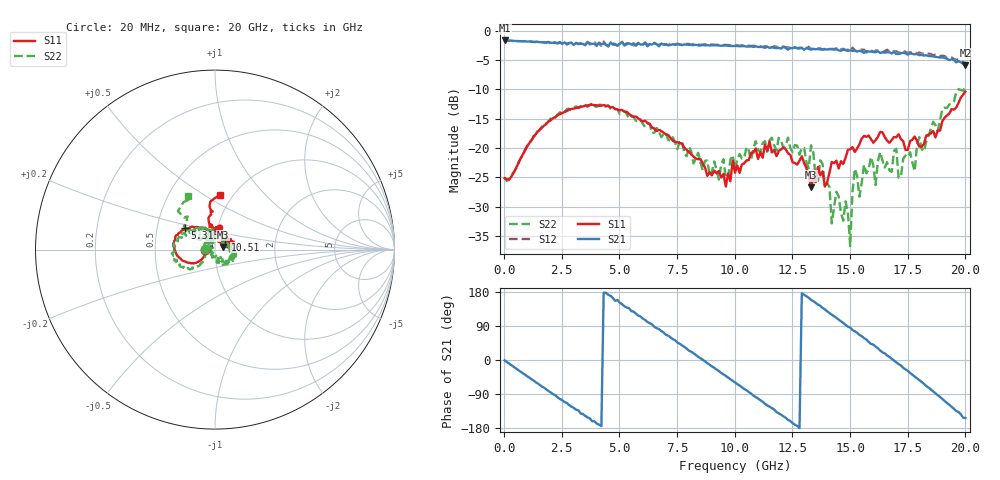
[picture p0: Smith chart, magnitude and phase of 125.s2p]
!Agilent Technologies,N5230A,US43500223,A.07.50.48
!Agilent N5230A: A.07.50.48
!Date: Sunday, September 13, 2015 22:02:00
!Correction: S11(Full 2 Port(1,2))
!S21(Full 2 Port(1,2))
!S12(Full 2 Port(1,2))
!S22(Full 2 Port(1,2))
!S2P File: Measurements: S11, S21, S12, S22:
# Hz S  dB  R 50
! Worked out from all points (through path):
!   201 points, 20 MHz to 20 GHz, reference 50 ohm
!   highest |S21| = -1.65 dB at 20 MHz (marker M1); lowest = -5.9 dB at 20 GHz (marker M2)
!   group delay of S21, straight-line fit = 120 ps
!   lowest |S11| = -26.7 dB at 13.31 GHz (marker M3), VSWR 1.10, Z = 54.6 + j1.55 ohm
!   |S11| at or under -10 dB: start of sweep to end of sweep
!   |S22| runs from -36.7 to -9.6 dB; largest |S21 - S12| = 0.051
!   S11 on the Smith chart (normalised r, x): 20 MHz: 0.89, +0.00; 5.315 GHz: 0.70, +0.17; 10.51 GHz: 1.11, +0.13; 20 GHz: 0.87, +0.58
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2e7  -25.12 179.9  -1.65 -1.0  -1.67 -1.0  -24.97 179.0
1.9181e9  -15.48 -154.2  -1.90 -81.6  -1.91 -82.0  -15.49 -140.4
3.4166e9  -12.92 177.7  -2.25 -142.6  -2.51 -141.9  -12.62 -164.9
5.3147e9  -13.80 144.6  -2.32 138.5  -2.12 140.1  -14.17 151.4
6.7133e9  -16.90 120.6  -2.66 81.6  -2.47 80.8  -17.12 118.1
8.3117e9  -21.80 101.3  -2.38 13.4  -2.26 13.2  -21.71 88.6
1.001e10  -24.20 58.4  -2.59 -59.2  -2.45 -59.8  -23.57 6.5
1.05095e10  -22.11 45.7  -2.71 -80.2  -2.59 -81.7  -19.81 2.8
1.21079e10  -19.90 15.4  -2.75 -148.8  -2.67 -148.8  -19.99 -26.8
1.33067e10  -26.68 17.9  -3.21 158.9  -3.12 158.1  -19.55 -49.8
1.34066e10  -24.92 31.4  -3.10 155.4  -3.06 154.7  -20.75 -68.6
1.41059e10  -24.21 60.8  -3.15 123.8  -3.11 122.0  -26.61 -110.8
1.42058e10  -22.38 58.2  -3.16 119.7  -3.09 120.1  -32.84 -138.3
1.48052e10  -21.63 68.0  -3.33 92.7  -3.28 91.5  -29.08 -163.7
1.5005e10  -20.21 62.4  -3.35 85.3  -3.44 86.0  -36.72 139.6
1.52048e10  -20.66 65.4  -3.41 75.7  -3.28 73.7  -23.53 153.5
1.54046e10  -19.36 73.4  -3.41 66.3  -3.20 68.1  -28.29 102.7
1.59041e10  -18.48 74.6  -3.54 42.4  -3.29 43.6  -21.53 110.2
1.67033e10  -19.10 83.7  -3.67 8.1  -3.57 6.1  -23.78 113.6
1.78022e10  -18.02 87.0  -4.03 -44.0  -3.66 -45.8  -23.93 141.8
1.85015e10  -17.51 96.8  -4.34 -77.3  -3.94 -80.1  -16.73 147.0
2e10  -10.38 85.1  -5.86 -153.4  -5.61 -156.8  -9.55 117.0
